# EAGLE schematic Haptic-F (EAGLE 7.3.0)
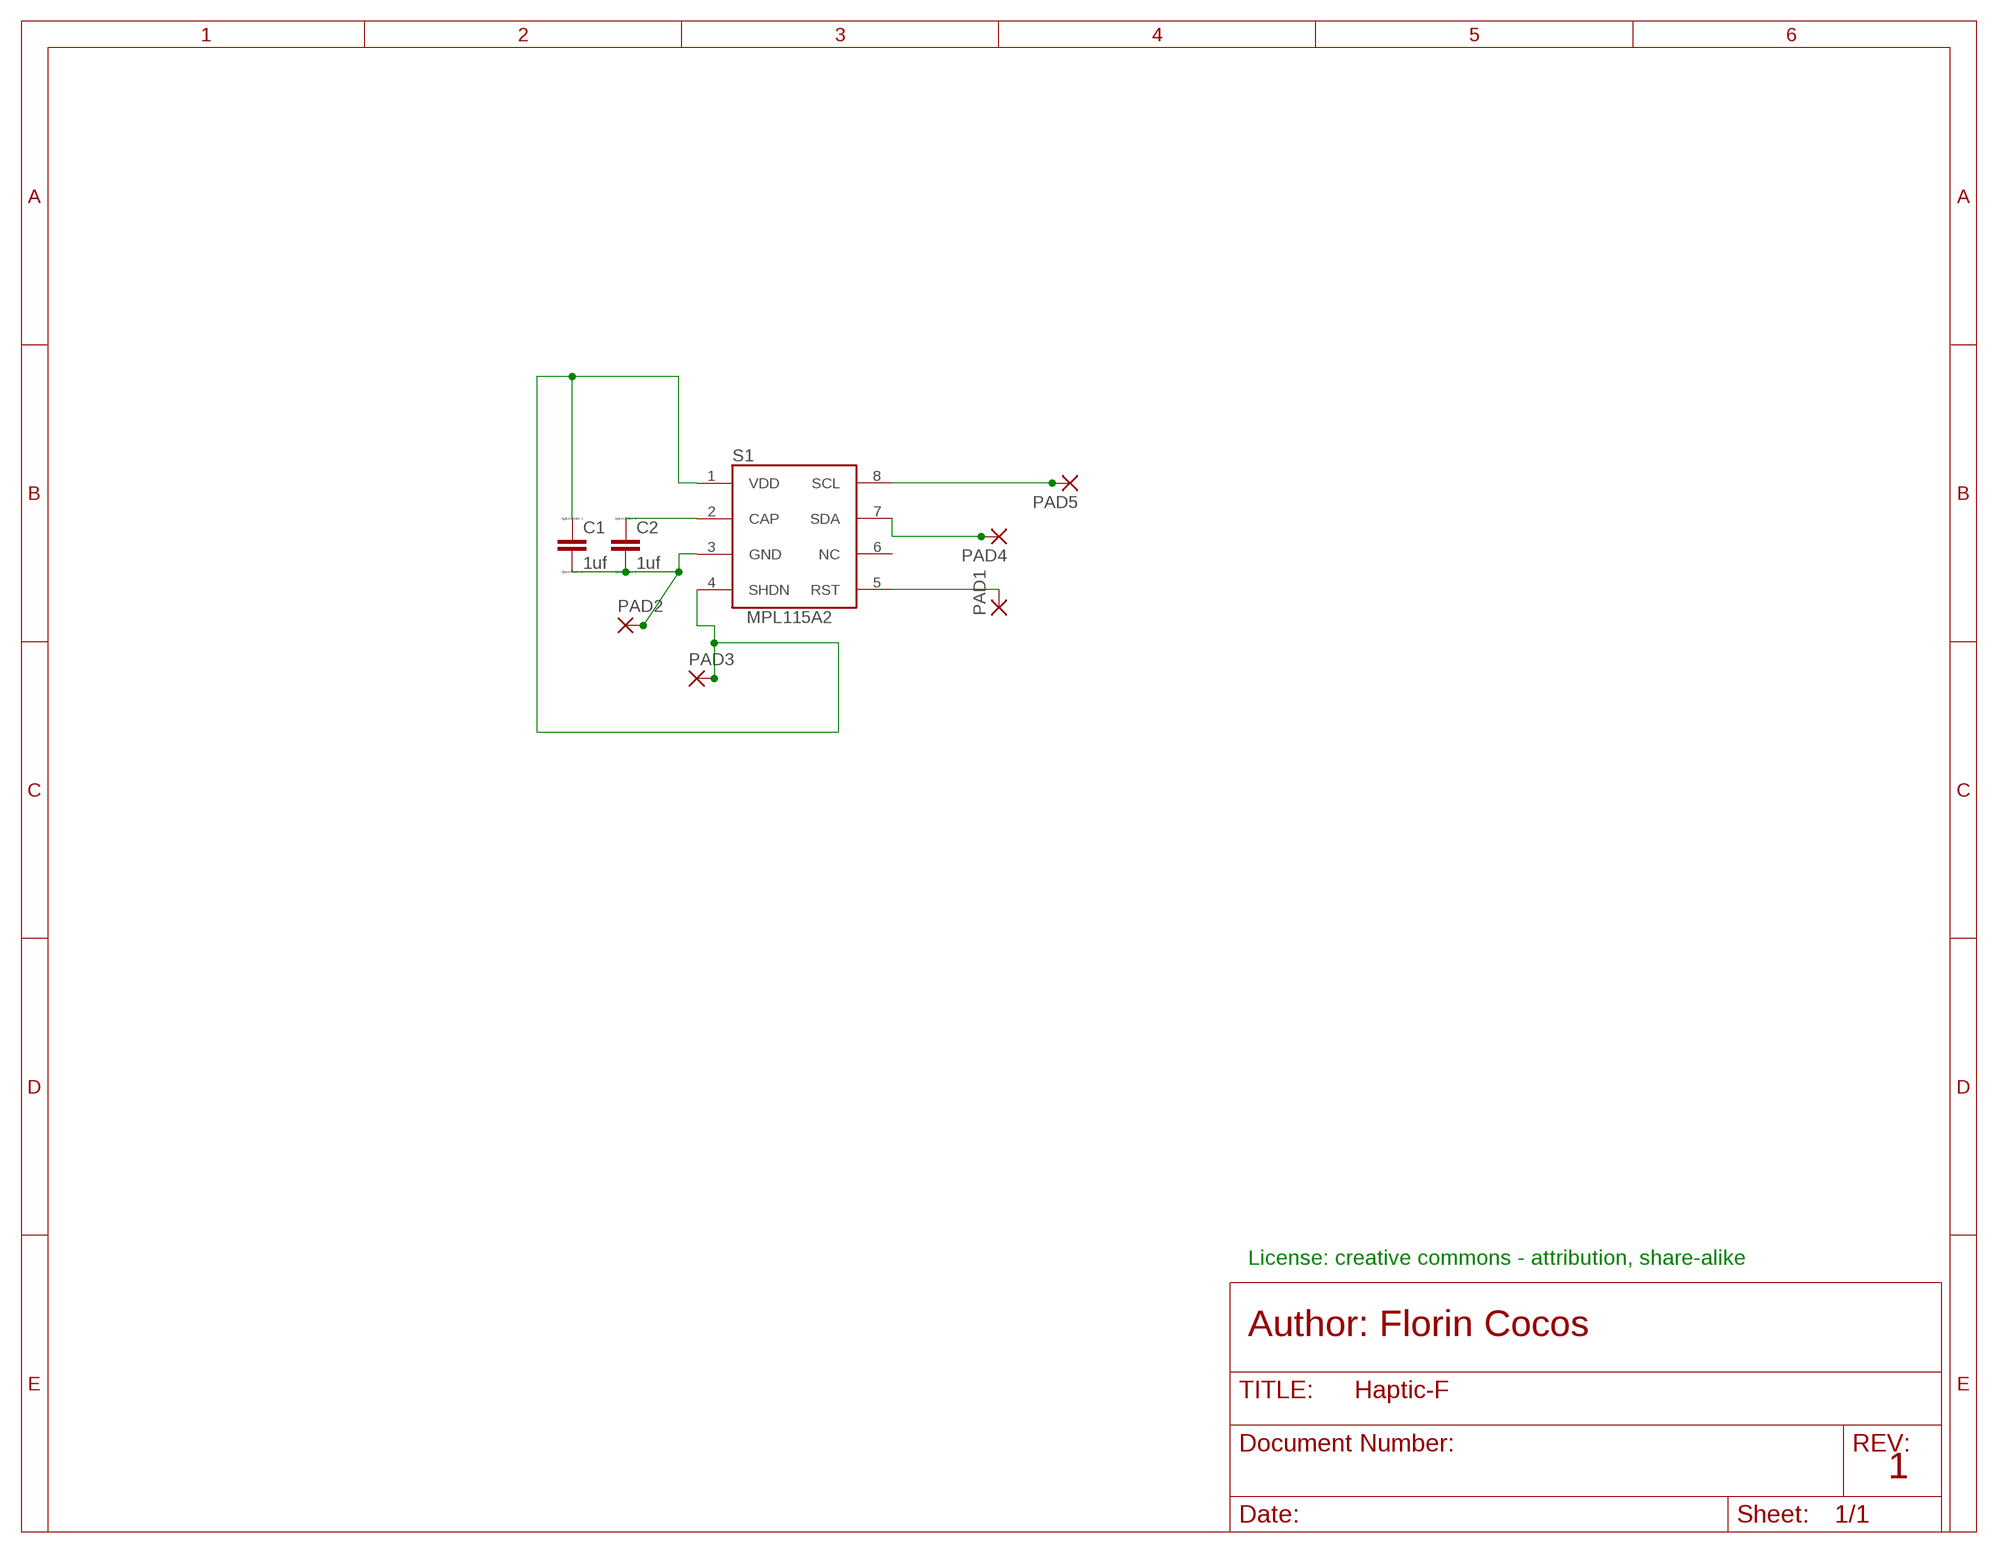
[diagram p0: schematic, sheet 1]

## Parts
C1  1uf  CC0402  [C0402]
C2  1uf  CC0402  [C0402]
PAD1  1,6/0,8  [1,6/0,8]
PAD2  1,6/0,8  [1,6/0,8]
PAD3  1,6/0,8  [1,6/0,8]
PAD4  1,6/0,8  [1,6/0,8]
PAD5  1,6/0,8  [1,6/0,8]
S1  MPL115A2  [LGA8]

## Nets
CAP: C2.1 S1.2(CAP)
GND: C1.2 C2.2 PAD2.1(P) S1.3(GND)
RST: PAD1.1(P) S1.5(RST)
SCL: PAD5.1(P) S1.8(SCL)
SDA: PAD4.1(P) S1.7(SDA)
VDD: C1.1 PAD3.1(P) S1.1(VDD) S1.4(SHDN)
Unconnected: S1.6(NC)

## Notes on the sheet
- License: creative commons - attribution, share-alike
- Author: Florin Cocos
- 1

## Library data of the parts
C1 C2 = eagle-ltspice:C: CAPACITOR, European symbol; SPICEMODEL: NONE; SPICEPREFIX: C
PAD1-PAD5 = wirepad:1,6/0,8: THROUGH-HOLE PAD
S1 = Youritronics:MPL115A2: MPL115A2 employs a MEMS pressure sensor with a conditioning IC to provide accurate pressure measurement from 50 to 115 kPa. An integrated ADC provides digitized temperature and pressure sensor outputs via an I2C port. Calibration Data is stored in internal ROM. Utilizing raw sensor output, the host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

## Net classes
0 default: width 0.127 mm, drill 0.508 mm, clearance 0.254 mm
